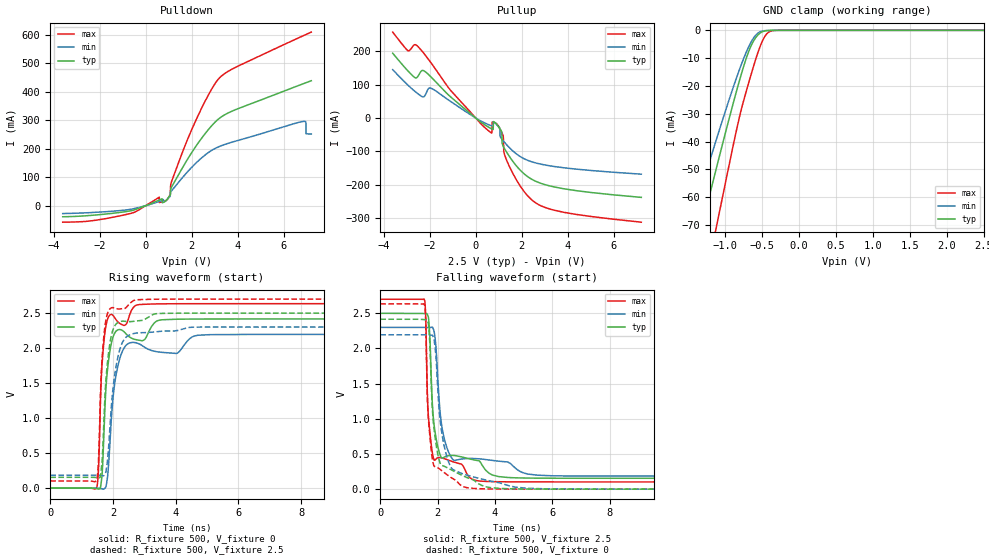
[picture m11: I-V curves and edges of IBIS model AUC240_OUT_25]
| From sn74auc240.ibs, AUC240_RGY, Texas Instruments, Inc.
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[Model]   AUC240_OUT_25
Model_type  3-state
Enable   Active-Low
Vref =   0
Rref =   500
Cref =   30p
Vmeas =   1.25
| variable   typ   min   max
C_comp   5.41pF   4.88pF   5.67pF
| C_pullup   7.85pF   4.33pF   12.14pF
| C_pulldown   6.87pF   4.92pF   15.47pF
| C_tri-state   5.41pF   4.88pF   5.67pF
[Temperature Range]   40   100   -40
| Ambient temperature   25   85   -40
[Voltage range]   2.5   2.3   2.7
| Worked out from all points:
|   slope of the pulldown table from 0 to 0.375 V, typ, clamps not added: 30.7 ohm
|   slope of the pullup table from 0 to 0.375 V, typ, clamps not added: 19.3 ohm
|   GND clamp passes 1 mA (typ) near -0.53 V on its own axis
|   rising waveform, R_fixture 500, V_fixture 0: 20-80 % time 209ps typ, 287ps min, 155ps max; typ from 0 V to 2.42 V
|   falling waveform, R_fixture 500, V_fixture 2.5: 20-80 % time 253ps typ, 343ps min, 181ps max; typ from 2.5 V to 0.154 V
|   rising waveform, R_fixture 500, V_fixture 2.5: 20-80 % time 209ps typ, 296ps min, 155ps max; typ from 0.154 V to 2.5 V
|   falling waveform, R_fixture 500, V_fixture 0: 20-80 % time 271ps typ, 375ps min, 185ps max; typ from 2.42 V to 0 V
[GND Clamp]
| AUC240_OUT_25
|   Voltage   I(typ)   I(min)   I(max)
-3.6V     -319.1mA   -267.5mA   -389.1mA
-1.46V    -86.02mA   -69.12mA   -115.2mA
-1.35V    -74.21mA   -59.38mA   -100.9mA
-1.295V   -68.33mA   -54.55mA   -93.77mA
-1.105V   -48.23mA   -38.17mA   -69.07mA
-840mV    -21.37mA   -16.68mA   -35.22mA
-725mV    -11.01mA   -8.595mA   -23.02mA
-625mV    -4.333mA   -3.195mA   -13.84mA
-525mV    -969.3uA   -537.7uA   -5.77mA
-435mV    -119.4uA   -67.11uA   -1.249mA
-325mV    -4.914uA   -5.524uA   -43.94uA
2.5V      1.045nA    235.6nA    1.469nA
[Pulldown]
| AUC240_OUT_25
|   Voltage   I(typ)   I(min)   I(max)
-3.6V     -38.75mA   -27.46mA   -57.79mA
-1.145V   -23.84mA   -17.22mA   -36.09mA
590mV     19.92mA    14.98mA    30.03mA
600mV     20.28mA    15.25mA    11.17mA
910mV     19.98mA    20.14mA    19.19mA
1.14V     67.22mA    53.43mA    87.3mA
1.925V    176.6mA    128mA      252.2mA
3.16V     303.8mA    206.4mA    444.2mA
6.825V    427.5mA    295.7mA    595.8mA
6.965V    431.8mA    292.9mA    601mA
6.97V     431.9mA    252.6mA    601.2mA
7.2V      438.8mA    251.8mA    609.5mA
[Pullup]
| AUC240_OUT_25
|   Voltage   I(typ)   I(min)   I(max)
-3.6V     193.7mA    144.6mA    256.9mA
-2.935V   140.5mA    97.95mA    200.9mA
-2.49V    125.8mA    71.54mA    212.7mA
-1.91V    120.8mA    88.21mA    162.4mA
445mV     -22.7mA    -16.54mA   -31.6mA
945mV     -21.56mA   -22.07mA   -19.39mA
1.14V     -42.13mA   -63.07mA   -43.86mA
1.19V     -82.98mA   -67.32mA   -51.19mA
1.235V    -89.26mA   -71.06mA   -103.2mA
1.455V    -113.7mA   -87.91mA   -143.1mA
2.52V     -186.4mA   -132.8mA   -249.6mA
7.2V      -237.6mA   -168.2mA   -311.9mA
[Ramp]
| AUC240_OUT_25
| variable   typ   min   max
dV/dt_r   1.46/2.13E-10   1.33/2.91E-10   1.59/1.57E-10
dV/dt_f   1.41/2.54E-10   1.27/3.49E-10   1.56/1.81E-10
R_load = 500
[Rising Waveform]
| AUC240_OUT_25
R_fixture =   500
C_fixture =   0
L_fixture =   0
V_fixture =   0
V_fixture_min = 0
V_fixture_max = 0
|   Time   V(typ)   V(min)   V(max)
0s        13.61nV    40.86nV    2.087nV
1.485ns   -7.106mV   406.7uV    14.16mV
1.54ns    -12.34mV   -781.8uV   292.3mV
1.65ns    186.2mV    -9.51mV    1.76V
1.795ns   1.552V     66.57mV    2.361V
2.15ns    2.259V     1.734V     2.377V
2.77ns    2.117V     2.071V     2.616V
4.01ns    2.412V     1.924V     2.633V
5.1ns     2.415V     2.192V     2.634V
34.99ns   2.416V     2.195V     2.634V
[Falling Waveform]
| AUC240_OUT_25
R_fixture =   500
C_fixture =   0
L_fixture =   0
V_fixture =   2.5
V_fixture_min = 2.3
V_fixture_max = 2.7
|   Time   V(typ)   V(min)   V(max)
0s        2.5V       2.3V       2.7V
1.53ns    2.496V     2.299V     2.703V
1.585ns   2.496V     2.299V     2.437V
1.67ns    2.454V     2.298V     1.083V
1.865ns   948.2mV    2.257V     424.1mV
2.1ns     472.4mV    1.035V     447.8mV
2.315ns   470.7mV    596.5mV    421.8mV
3.355ns   408.7mV    434mV      122.2mV
4.93ns    159.3mV    240.9mV    103.4mV
34.99ns   154.5mV    184.4mV    102.7mV
[Rising Waveform]
| AUC240_OUT_25
R_fixture =   500
C_fixture =   0
L_fixture =   0
V_fixture =   2.5
V_fixture_min = 2.3
V_fixture_max = 2.7
|   Time   V(typ)   V(min)   V(max)
0s        154.5mV    184.4mV    102.6mV
1.485ns   148.9mV    184.7mV    121.6mV
1.54ns    145.9mV    183.7mV    427mV
1.64ns    326.5mV    178.6mV    1.76V
1.79ns    1.635V     276.1mV    2.436V
1.99ns    2.249V     1.38V      2.578V
2.15ns    2.363V     1.859V     2.559V
2.36ns    2.384V     2.126V     2.563V
2.715ns   2.386V     2.213V     2.688V
34.99ns   2.5V       2.3V       2.7V
[Falling Waveform]
| AUC240_OUT_25
R_fixture =   500
C_fixture =   0
L_fixture =   0
V_fixture =   0
V_fixture_min = 0
V_fixture_max = 0
|   Time   V(typ)   V(min)   V(max)
0s        2.416V     2.195V     2.634V
1.53ns    2.411V     2.194V     2.634V
1.58ns    2.409V     2.194V     2.42V
1.64ns    2.394V     2.192V     1.314V
1.69ns    2.3V       2.191V     931.1mV
1.845ns   974.1mV    2.163V     366.5mV
2.09ns    365.8mV    965mV      280.2mV
2.275ns   316.8mV    528.4mV    220.8mV
3.02ns    165.3mV    199.1mV    21mV
34.99ns   30.09uV    827.3nV    13.48uV
